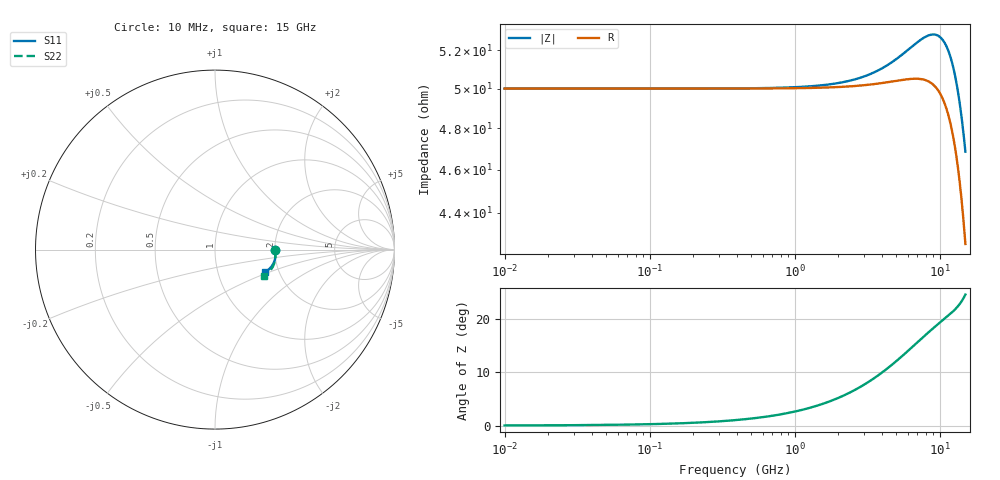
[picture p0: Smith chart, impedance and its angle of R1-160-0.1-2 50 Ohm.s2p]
!version-2
!date-03.2021
# MHz S RI R 50
!Freq ReS11 ImS11 ReS21 ImS21 ReS12 ImS12 ReS22 ImS22
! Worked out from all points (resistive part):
!   751 points, 10 MHz to 15 GHz, reference 50 ohm
!   read as one part in series: R = 50 ohm at 70 MHz
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10  0.3333 -3.8e-05  0.6667 -0.00022  0.6667 -0.00022  0.3333 -5.24e-05
70  0.3333 -0.000266  0.6667 -0.00154  0.6667 -0.00154  0.3333 -0.000367
1250  0.3336 -0.00482  0.6659 -0.0275  0.6659 -0.0275  0.3336 -0.00662
2510  0.3343 -0.0101  0.6635 -0.0548  0.6635 -0.0548  0.3342 -0.0137
3810  0.3352 -0.0164  0.6596 -0.0823  0.6596 -0.0823  0.3351 -0.022
5010  0.3361 -0.0234  0.655 -0.1067  0.655 -0.1067  0.3359 -0.0308
5650  0.3364 -0.0277  0.6522 -0.1193  0.6522 -0.1193  0.3361 -0.036
6270  0.3365 -0.0322  0.6494 -0.1312  0.6494 -0.1312  0.3361 -0.0415
6890  0.3364 -0.0371  0.6465 -0.1428  0.6465 -0.1428  0.3359 -0.0474
7510  0.336 -0.0423  0.6437 -0.1541  0.6437 -0.1541  0.3353 -0.0536
8170  0.3352 -0.0484  0.6407 -0.1658  0.6407 -0.1658  0.3342 -0.0608
8810  0.3338 -0.0547  0.6379 -0.1768  0.6379 -0.1768  0.3326 -0.0681
9430  0.332 -0.0612  0.6354 -0.1873  0.6354 -0.1873  0.3305 -0.0755
10010  0.3297 -0.0676  0.6333 -0.1969  0.6333 -0.1969  0.328 -0.0828
10650  0.3265 -0.0749  0.6313 -0.2074  0.6313 -0.2074  0.3244 -0.0911
11290  0.3225 -0.0825  0.6298 -0.2178  0.6298 -0.2178  0.32 -0.0995
11910  0.3178 -0.0899  0.6287 -0.2279  0.6287 -0.2279  0.3148 -0.1078
12510  0.3123 -0.0972  0.6281 -0.2379  0.6281 -0.2379  0.3089 -0.1159
13150  0.3055 -0.1049  0.628 -0.2487  0.628 -0.2487  0.3016 -0.1243
13770  0.2979 -0.1122  0.6283 -0.2596  0.6283 -0.2596  0.2935 -0.1323
14350  0.2899 -0.1187  0.6291 -0.2703  0.6291 -0.2703  0.285 -0.1394
15000  0.2799 -0.1256  0.6305 -0.2829  0.6305 -0.2829  0.2745 -0.1468
